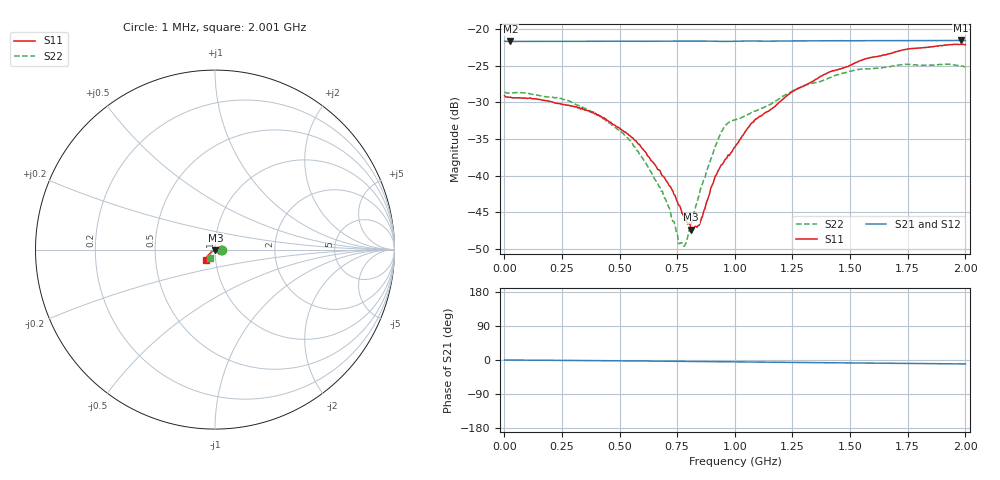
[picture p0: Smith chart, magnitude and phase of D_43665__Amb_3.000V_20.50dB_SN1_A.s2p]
! device id: 43665_
! dir: \\malibu\benchdata\1_engineers\tn_data\43665_75ohm\new\sparar\43665_\amb\3p000v\20p50db
! Serial: 1
! Insertion: A
! Temp: Amb
! VDD: 3.000V
! Attenuation Step: 20.50dB
! IDD: 1.450588e+00mA
! FILE NAME
! DATE 03-27-2009 08:38:22
! CORRECTED  DATA
#  Hz  S  RI  R  75
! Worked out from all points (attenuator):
!   401 points, 1 MHz to 2.001 GHz, reference 75 ohm
!   highest |S21| = -21.54 dB at 1.981 GHz (marker M1); lowest = -21.7 dB at 26 MHz (marker M2)
!   lowest |S11| = -47.4 dB at 811 MHz (marker M3), VSWR 1.01, Z = 75.3 - j0.551 ohm
!   |S11| at or under -10 dB: start of sweep to end of sweep
!   |S22| runs from -49.6 to -24.8 dB; largest |S21 - S12| = 0.00041
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1000000  0.0351 -0.000483  0.0828 -0.000117  0.0827 -7.34e-05  0.0373 -0.000374
2.6e7  0.0343 -1.72e-06  0.0824 -0.000146  0.0825 -0.000168  0.0366 0.000731
2.36e8  0.0311 0.00162  0.0825 -0.0014  0.0826 -0.00134  0.0329 0.00814
3.36e8  0.0289 0.00192  0.0826 -0.00206  0.0826 -0.00198  0.0275 0.0104
5.26e8  0.0198 0.0014  0.0826 -0.00339  0.0827 -0.00326  0.016 0.00953
6.01e8  0.0152 0.000604  0.0825 -0.00385  0.0826 -0.00372  0.0096 0.00896
6.71e8  0.0109 -0.000739  0.0827 -0.00433  0.0827 -0.00415  0.00563 0.00629
7.11e8  0.00867 -0.00167  0.0827 -0.00462  0.0828 -0.00446  0.00349 0.00514
7.66e8  0.00529 -0.00269  0.0827 -0.00513  0.0828 -0.00493  -0.00119 0.00328
7.86e8  0.00391 -0.00309  0.0827 -0.00528  0.0828 -0.00513  -0.00287 0.00183
8.11e8  0.00222 -0.00366  0.0828 -0.00557  0.0828 -0.00535  -0.00469 -7.04e-05
8.51e8  -0.000603 -0.00482  0.0827 -0.00592  0.0827 -0.00572  -0.0074 -0.0033
9.06e8  -0.00508 -0.0073  0.0825 -0.00646  0.0825 -0.00623  -0.0118 -0.00814
9.31e8  -0.00698 -0.00854  0.0823 -0.00658  0.0824 -0.00636  -0.0152 -0.0101
9.61e8  -0.00873 -0.00962  0.0822 -0.00659  0.0823 -0.00641  -0.0198 -0.00989
1.001e9  -0.0119 -0.0103  0.0824 -0.00664  0.0825 -0.00645  -0.0223 -0.00914
1.096e9  -0.0196 -0.0148  0.0826 -0.00778  0.0827 -0.0075  -0.0238 -0.0144
1.336e9  -0.0341 -0.0274  0.0828 -0.00958  0.083 -0.00931  -0.0299 -0.0304
1.521e9  -0.0439 -0.0388  0.0826 -0.0114  0.0829 -0.0111  -0.0327 -0.0411
1.671e9  -0.0485 -0.0477  0.0825 -0.0126  0.0828 -0.0125  -0.032 -0.0452
1.981e9  -0.0502 -0.0608  0.0824 -0.015  0.0826 -0.0151  -0.0282 -0.0486
2.001e9  -0.0497 -0.0606  0.0823 -0.0151  0.0824 -0.0152  -0.0278 -0.0479
